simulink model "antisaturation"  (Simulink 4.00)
settings: Solver=FixedStepDiscrete  StartTime=0.0  StopTime=10.5  FixedStep=0.01  RelTol=1e-3
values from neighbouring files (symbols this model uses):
  A = [1 -0.7846 -0.2154]    [antisat.m]    (also in antisat_old.m)
  Am = track_discr.den{1}    [antisat_old.m]
  B = [0 -0.03476 -0.1112]    [antisat.m]    (also in antisat_old.m)
  Bm = track_discr.num{1}    [antisat_old.m]
  Ps = [S(1) S(1)*p1]    [antisat.m]    (also in antisat_old.m = [S(1)/(1+p1) S(1)*p1/(1+p1)])
  Ts = 0.12    [antisat.m]    (also in antisat_old.m)
  Umax = 5    [antisat.m]    (also in antisat_old.m = 100)
  Umin = -5    [antisat.m]    (also in antisat_old.m = -100)
undefined symbols (not defined in the file or in its folder): R, S, T

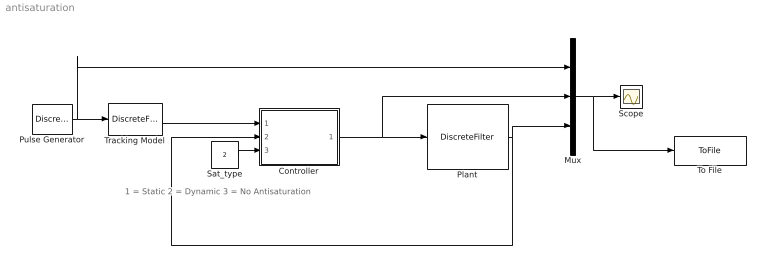
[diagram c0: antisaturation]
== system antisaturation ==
  note: 1 = Static 2 = Dynamic 3 = No Antisaturation
  Controller : Subsystem
  Mux : Mux  Inputs=3
  Plant : DiscreteFilter  Numerator=B  Denominator=A  SampleTime=Ts  Realization=auto
  Pulse Generator : DiscretePulseGenerator  PulseType=Sample-based  Amplitude=5  Period=80  PulseWidth=40  PhaseDelay=8  SampleTime=Ts
  Sat_type : Constant  Value=2
  Scope : Scope
  To File : ToFile  Filename=antisat_dyn2.mat  MatrixName=measures  SampleTime=Ts
  Tracking Model : DiscreteFilter  Numerator=Bm  Denominator=Am  SampleTime=Ts  Realization=auto
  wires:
  Plant/1 -> Controller/2(Y), Mux/3
  Controller/1(Command) -> Plant/1, Mux/2
  Pulse Generator/1 -> Tracking Model/1, Mux/1
  Tracking Model/1 -> Controller/1(YDes)
  Mux/1 -> Scope/1, To File/1
  Sat_type/1 -> Controller/3(Sat)

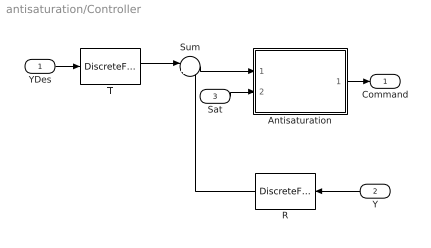
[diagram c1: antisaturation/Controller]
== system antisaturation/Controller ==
  YDes : Inport  Port=1  LatchInput=off
  Y : Inport  Orientation=left  Port=2  LatchInput=off
  Sat : Inport  Port=3  LatchInput=off
  Antisaturation : Subsystem
  R : DiscreteFilter  Orientation=left  Numerator=R  Denominator=1  SampleTime=Ts  Realization=auto
  Sum : Sum  Inputs=|+-  SaturateOnIntegerOverflow=on
  T : DiscreteFilter  Numerator=T  Denominator=1  SampleTime=Ts  Realization=auto
  Command : Outport  Port=1
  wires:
  T/1 -> Sum/1
  R/1 -> Sum/2
  Sum/1 -> Antisaturation/1(T*YDes-R*Y)
  YDes/1 -> T/1
  Y/1 -> R/1
  Antisaturation/1(Command) -> Command/1
  Sat/1 -> Antisaturation/2(Saturation type)

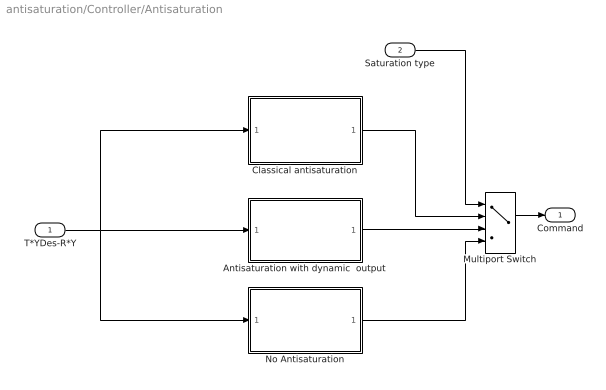
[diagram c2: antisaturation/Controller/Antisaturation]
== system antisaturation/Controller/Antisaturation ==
  T*YDes-R*Y : Inport  Port=1  LatchInput=off
  Saturation type : Inport  Port=2  LatchInput=off
  Antisaturation with dynamic  output : Subsystem
  Classical antisaturation : Subsystem
  Multiport Switch : MultiPortSwitch  Inputs=3
  No Antisaturation : Subsystem
  Command : Outport  Port=1
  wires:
  T*YDes-R*Y/1 -> Antisaturation with dynamic  output/1(T*YDes-R*Y), Classical antisaturation/1(T*YDes-R*Y), No Antisaturation/1(T*YDes-R*Y)
  Multiport Switch/1 -> Command/1
  Saturation type/1 -> Multiport Switch/1
  Classical antisaturation/1(Command) -> Multiport Switch/2
  Antisaturation with dynamic  output/1(Command) -> Multiport Switch/3
  No Antisaturation/1("Command ") -> Multiport Switch/4

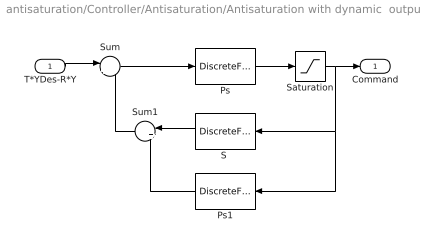
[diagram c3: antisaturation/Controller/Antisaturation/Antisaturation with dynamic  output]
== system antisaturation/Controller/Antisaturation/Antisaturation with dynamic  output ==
  T*YDes-R*Y : Inport  Port=1  LatchInput=off
  Ps : DiscreteFilter  Numerator=[1]  Denominator=Ps  SampleTime=Ts  Realization=auto
  Ps1 : DiscreteFilter  Orientation=left  Numerator=Ps  Denominator=1  SampleTime=Ts  Realization=auto
  "S " : DiscreteFilter  Orientation=left  Numerator=S  Denominator=1  SampleTime=Ts  Realization=auto
  Saturation : Saturate  UpperLimit=Umax  LowerLimit=Umin  LinearizeAsGain=on
  Sum : Sum  Inputs=|+-  SaturateOnIntegerOverflow=on
  Sum1 : Sum  Orientation=left  Inputs=|+-  SaturateOnIntegerOverflow=on
  Command : Outport  Port=1
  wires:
  Saturation/1 -> Command/1, "S "/1, Ps1/1
  Ps/1 -> Saturation/1
  Sum/1 -> Ps/1
  T*YDes-R*Y/1 -> Sum/1
  "S "/1 -> Sum1/1
  Ps1/1 -> Sum1/2
  Sum1/1 -> Sum/2

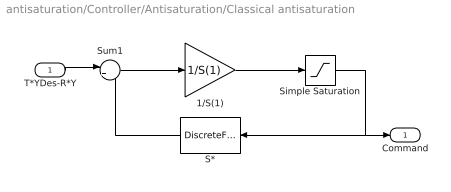
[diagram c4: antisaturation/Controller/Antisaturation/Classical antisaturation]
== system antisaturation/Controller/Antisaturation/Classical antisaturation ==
  T*YDes-R*Y : Inport  Port=1  LatchInput=off
  1/S(1) : Gain  Gain=1/S(1)  Multiplication=Element-wise(K.*u)  SaturateOnIntegerOverflow=on
  S* : DiscreteFilter  Orientation=left  Numerator=[0 S(2:end)]  Denominator=1  SampleTime=Ts  Realization=auto
  Simple Saturation : Saturate  UpperLimit=Umax  LowerLimit=Umin  LinearizeAsGain=on
  Sum1 : Sum  Inputs=|+-  SaturateOnIntegerOverflow=on
  Command : Outport  Port=1
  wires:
  Simple Saturation/1 -> S*/1, Command/1
  S*/1 -> Sum1/2
  Sum1/1 -> 1/S(1)/1
  1/S(1)/1 -> Simple Saturation/1
  T*YDes-R*Y/1 -> Sum1/1

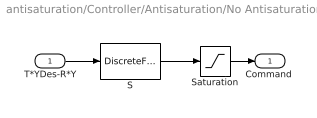
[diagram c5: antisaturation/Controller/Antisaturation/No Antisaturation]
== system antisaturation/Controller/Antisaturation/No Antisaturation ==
  T*YDes-R*Y : Inport  Port=1  LatchInput=off
  S : DiscreteFilter  Numerator=1  Denominator=S  SampleTime=Ts  Realization=auto
  Saturation : Saturate  UpperLimit=Umax  LowerLimit=Umin  LinearizeAsGain=on
  "Command " : Outport  Port=1
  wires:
  S/1 -> Saturation/1
  T*YDes-R*Y/1 -> S/1
  Saturation/1 -> "Command "/1
